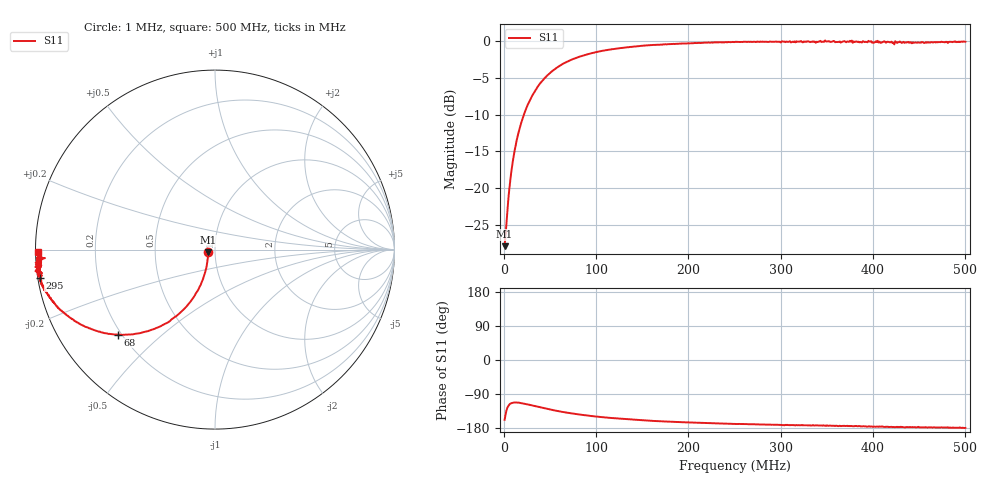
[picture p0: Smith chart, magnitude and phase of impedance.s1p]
# Hz S RI R 50.0
! written by SimSmith version 18.3b
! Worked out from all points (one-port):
!   500 points, 1 MHz to 500 MHz, reference 50 ohm
!   lowest |S11| = -27.9 dB at 1 MHz (marker M1), VSWR 1.08, Z = 46.4 - j1.42 ohm
!   |S11| at or under -10 dB: start of sweep to 21.89 MHz
!   S11 on the Smith chart (normalised r, x): 1 MHz: 0.93, -0.03; 68 MHz: 0.19, -0.37; 295 MHz: 0.01, -0.08; 500 MHz: 0.01, -0.01
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1000000  -0.0374 -0.0153
3000000  -0.0397 -0.0422
6000000  -0.0458 -0.086
8000000  -0.0516 -0.1148
1e7  -0.0597 -0.1418
1.5e7  -0.086 -0.2075
2.1e7  -0.1277 -0.2777
2.9e7  -0.1944 -0.3522
3.8e7  -0.2798 -0.414
5e7  -0.3939 -0.4589
6.4e7  -0.5125 -0.4747
6.8e7  -0.5398 -0.474
8.1e7  -0.6248 -0.4624
9.7e7  -0.7064 -0.435
1.26e8  -0.8099 -0.3772
1.61e8  -0.8854 -0.3122
1.89e8  -0.9178 -0.2681
2.51e8  -0.9669 -0.193
2.95e8  -0.9773 -0.1582
3.13e8  -0.9772 -0.1447
3.76e8  -0.9834 -0.1013
3.86e8  -0.9809 -0.0883
3.96e8  -0.9875 -0.0845
4.01e8  -0.9706 -0.0736
4.09e8  -0.9696 -0.0734
4.23e8  -0.9471 -0.0472
4.38e8  -0.9836 -0.0489
5e8  -0.9868 -0.0141
